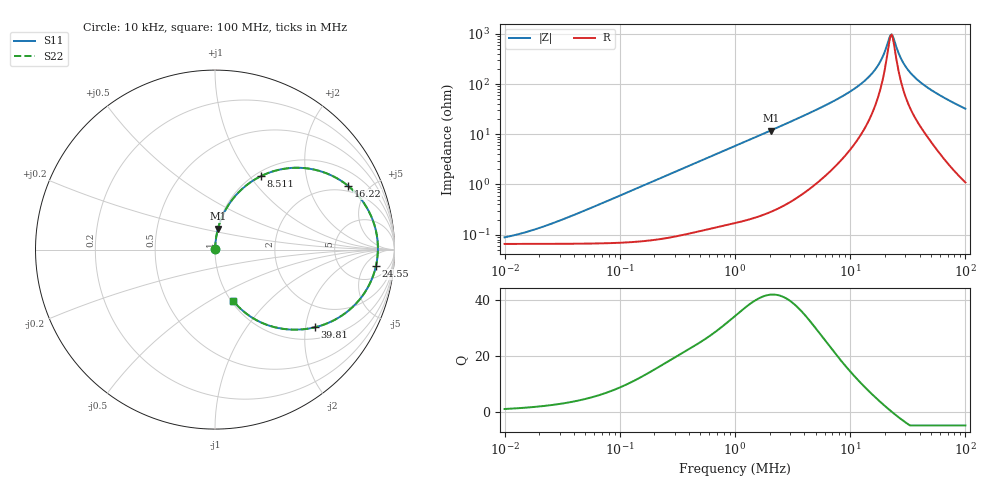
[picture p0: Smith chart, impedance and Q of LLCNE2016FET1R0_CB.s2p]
! LLCNE2016FET1R0_CB  S-PARAMETER MODEL  ( Standard Model )
! Model Generated by TAIYO YUDEN Corporation (http://www.ty-top.com)
! Version 1.0
! TAIYO YUDEN Control No. 200220
! Copyright(c) 2020 TAIYO YUDEN CO.,LTD. All Rights Reserved.
! Product Description (link to TY-COMPAS)
! https://ds.yuden.co.jp/TYCOMPAS/or/detail?pn=LLCNE2016FET1R0MCB&u=M
! Products Name : Inductors
! Characteristics :
!  Inductance : 1.0 [uH] , SRF(min) : - [Hz] , DC Resistance(max) : 70 [mOhm]
!  Rated Current : Saturation  2.8 [A] (dL = 30 [%]), Temp Rise  2.3 [A] (dT = 40 [degC])
!  Case Size : 2.0 x 1.6 / 0.079 x 0.063 [mm/inch] , Thickness : 0.65 / 0.026 [mm/inch]
!  (Conditions: Temperature = 25 [degC] , DC Bias Current = 0 [A])
! External Node Assignments :
!  1  o---GGG---o  2
! GND o---------o GND
! Frequency Range : 10kHz  -  100MHz  [ 402 STEP ]
# MHz S RI R 50
! Freq[MHz].  S11 Real  S11 Imag  S21 Real  S21 Imag  S12 Real  S12 Imag  S22 Real  S22 Imag
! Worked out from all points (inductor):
!   401 points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, 10 kHz to 100 MHz, reference 50 ohm
!   read as one part in series: L = 948 nH near 33.11 kHz
!   highest Q = 42 at 2.042 MHz (marker M1), where L = 928 nH
!   self-resonance near 22.8 MHz
!   S11 on the Smith chart (normalised r, x): 10 kHz: 1.00, +0.00; 8.511 MHz: 1.06, +1.14; 16.22 MHz: 1.68, +3.67; 24.55 MHz: 10, -10; 39.81 MHz: 1.31, -2.25; 100 MHz: 1.02, -0.65
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0.01  0.000653 0.000595  0.9993 -0.000595  0.9993 -0.000595  0.000653 0.000595
0.019498  0.000655 0.00116  0.9993 -0.00116  0.9993 -0.00116  0.000655 0.00116
0.046774  0.000668 0.00278  0.9993 -0.00278  0.9993 -0.00278  0.000668 0.00278
0.218776  0.000975 0.013  0.999 -0.013  0.999 -0.013  0.000975 0.013
1  0.00506 0.0579  0.9949 -0.0579  0.9949 -0.0579  0.00506 0.0579
2.041738  0.0167 0.1168  0.9833 -0.1168  0.9833 -0.1168  0.0167 0.1168
4.677351  0.0807 0.2569  0.9193 -0.2569  0.9193 -0.2569  0.0807 0.2569
6.456542  0.1513 0.3381  0.8487 -0.3381  0.8487 -0.3381  0.1513 0.3381
8.51138  0.2575 0.41  0.7425 -0.41  0.7425 -0.41  0.2575 0.41
12.30269  0.4995 0.454  0.5005 -0.454  0.5005 -0.454  0.4995 0.454
16.2181  0.7409 0.3555  0.2591 -0.3555  0.2591 -0.3555  0.7409 0.3555
19.05461  0.8571 0.2133  0.1429 -0.2133  0.1429 -0.2133  0.8571 0.2133
21.87762  0.9054 0.0516  0.0946 -0.0516  0.0946 -0.0516  0.9054 0.0516
22.90868  0.9076 -0.00573  0.0924 0.00573  0.0924 0.00573  0.9076 -0.00573
24.54709  0.8971 -0.0905  0.1029 0.0905  0.1029 0.0905  0.8971 -0.0905
26.91535  0.8598 -0.1952  0.1402 0.1952  0.1402 0.1952  0.8598 -0.1952
29.51209  0.8014 -0.2834  0.1986 0.2834  0.1986 0.2834  0.8014 -0.2834
33.88442  0.6913 -0.3775  0.3087 0.3775  0.3087 0.3775  0.6913 -0.3775
39.81072  0.556 -0.433  0.444 0.433  0.444 0.433  0.556 -0.433
48.97788  0.4005 -0.4441  0.5995 0.4441  0.5995 0.4441  0.4005 -0.4441
63.09573  0.2536 -0.4045  0.7464 0.4045  0.7464 0.4045  0.2536 -0.4045
100  0.103 -0.2875  0.897 0.2875  0.897 0.2875  0.103 -0.2875
